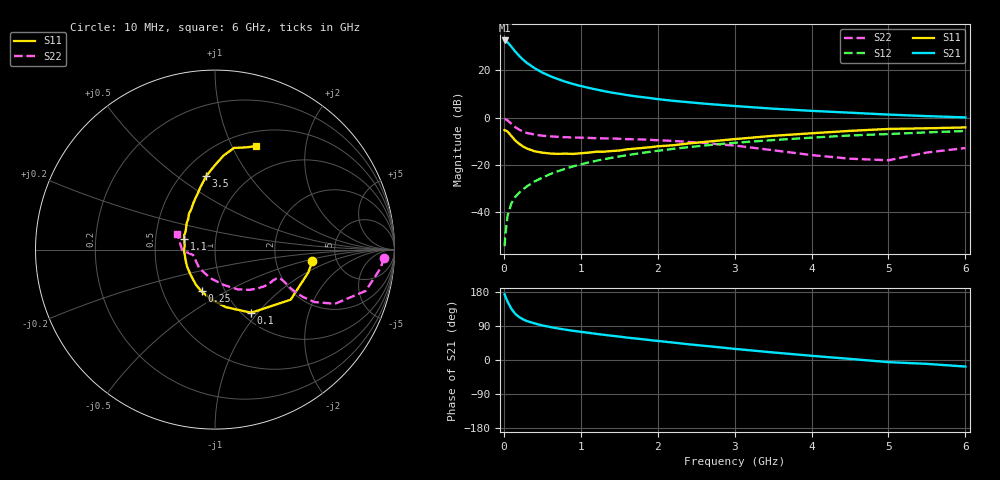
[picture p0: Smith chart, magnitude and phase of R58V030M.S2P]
! SIEMENS Small Signal Semiconductors
! BFR183
! Si NPN RF Bipolar Junction Transistor in SOT23
! VCE = 8 V  IC = 30 mA
! Common Emitter S-Parameters:  May  1996
# GHz  S  MA  R  50
!  f  S11  S21  S12  S22
! GHz  MAG  ANG  MAG  ANG  MAG  ANG  MAG  ANG
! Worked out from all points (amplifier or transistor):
!   36 points, 10 MHz to 6 GHz, reference 50 ohm
!   highest |S21| = 32.7 dB at 10 MHz (marker M1)
!   |S21| within 3 dB of that: start of sweep to 106.9 MHz
!   unconditionally stable (mu >= 1): 499.3 MHz to 2.469 GHz
!   at 250 MHz: K = 0.85, MSG = 27.4 dB, |S12| = -30.3 dB
!   at 1.4 GHz: K = 1.04, MAG = 12.6 dB, |S12| = -17.0 dB
!   at 6 GHz: K = 0.90, MSG = 2.9 dB, |S12| = -5.7 dB
!   S11 on the Smith chart (normalised r, x): 10 MHz: 3.28, -0.61; 100 MHz: 1.10, -0.93; 250 MHz: 0.78, -0.38; 1.1 GHz: 0.70, +0.08; 3.5 GHz: 0.65, +0.64; 6 GHz: 0.66, +1.25
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0.01  0.5458 -6.9  43.1 173.5  0.0019 84.4  0.9438 -2.8
0.02  0.5353 -13.8  42.52 168.0  0.0034 78.3  0.9273 -6.5
0.05  0.5056 -33.5  39.17 153.3  0.0087 76.7  0.871 -15.3
0.1  0.4056 -60.1  31.52 134.5  0.0156 71.6  0.7335 -24.3
0.15  0.3264 -79.3  24.93 121.4  0.0212 69.8  0.6268 -27.8
0.2  0.2789 -94.2  20.33 113.3  0.0258 70.3  0.5561 -28.3
0.25  0.2445 -107.9  16.89 107.2  0.0305 70.2  0.5066 -27.8
0.3  0.2219 -119.0  14.43 102.7  0.0351 71.7  0.4746 -27.1
0.4  0.1941 -135.1  11.15 96.6  0.0446 72.4  0.4372 -25.5
0.5  0.1815 -149.6  9.015 91.2  0.0536 73.2  0.4146 -24.4
0.6  0.1741 -160.0  7.599 87.2  0.0635 73.0  0.4018 -24.0
0.7  0.171 -170.8  6.577 83.4  0.073 72.8  0.3931 -23.9
0.8  0.1731 -178.6  5.768 80.1  0.083 72.0  0.3856 -24.2
0.9  0.1704 173.3  5.153 77.1  0.0929 71.5  0.38 -24.6
1.1  0.1816 161.3  4.285 71.8  0.1123 70.1  0.3725 -26.7
1.3  0.1904 151.1  3.647 66.5  0.1317 68.1  0.3639 -28.6
1.6  0.2133 138.0  3.006 59.2  0.1605 65.1  0.3509 -32.7
2.2  0.2601 120.7  2.274 46.0  0.2181 58.6  0.3219 -42.6
3.5  0.4122 96.9  1.549 19.9  0.3353 42.0  0.2042 -75.6
4.5  0.5251 84.9  1.273 2.9  0.419 29.6  0.1351 -131.1
5.5  0.5955 73.0  1.078 -10.2  0.4883 18.3  0.1829 -179.0
6  0.6214 68.2  1.012 -17.3  0.5211 10.9  0.2276 157.4
